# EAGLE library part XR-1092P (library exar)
EQUALIZER DISPLAY/FILTER/MULTIPLEXER
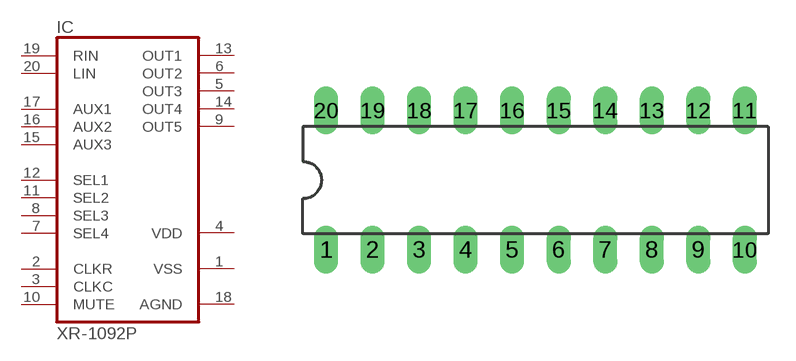
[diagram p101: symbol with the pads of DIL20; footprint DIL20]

Designator prefix IC

## XR-1092P (OC_FARNELL: unknown; OC_NEWARK: unknown)  [DIL20]
1  VSS  pwr
2  CLKR  in
3  CLKC  in
4  VDD  pwr
5  OUT3  out
6  OUT2  out
7  SEL4  in
8  SEL3  in
9  OUT5  out
10  MUTE  in
11  SEL2  in
12  SEL1  in
13  OUT1  out
14  OUT4  out
15  AUX3  in
16  AUX2  in
17  AUX1  in
18  AGND  pwr
19  RIN  in
20  LIN  in

## Footprint DIL20 (pad centres in mm)
Dual In Line Package
drill 0.813 long: 1 -11.43,-3.81; 2 -8.89,-3.81; 3 -6.35,-3.81; 4 -3.81,-3.81; 5 -1.27,-3.81; 6 1.27,-3.81; 7 3.81,-3.81; 8 6.35,-3.81; 9 8.89,-3.81; 10 11.43,-3.81; 11 11.43,3.81; 12 8.89,3.81; 13 6.35,3.81; 14 3.81,3.81; 15 1.27,3.81; 16 -1.27,3.81; 17 -3.81,3.81; 18 -6.35,3.81; 19 -8.89,3.81; 20 -11.43,3.81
